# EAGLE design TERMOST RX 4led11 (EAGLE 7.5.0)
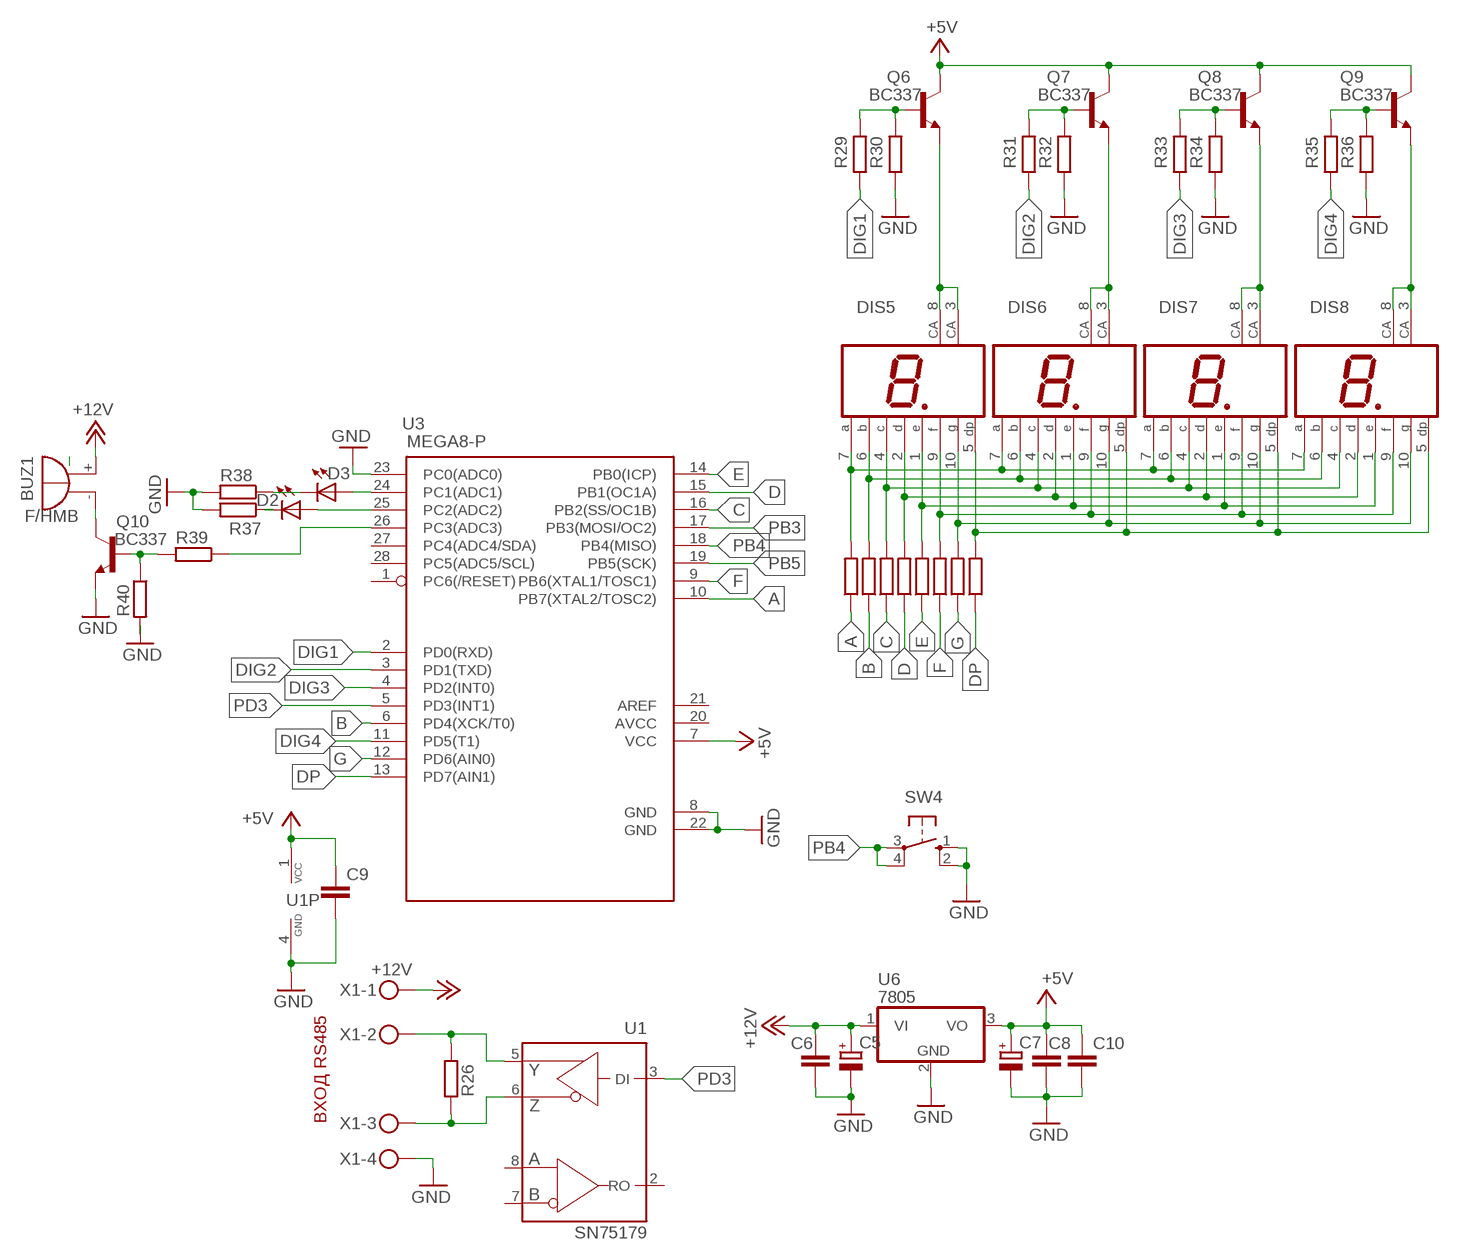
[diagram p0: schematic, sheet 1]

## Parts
BUZ1  F/HMB  [F/HMB]
C5  CPOL-EUE2.5-5  [E2,5-5]
C6  C-EUC1206  [C1206]
C7  CPOL-EUE2.5-5  [E2,5-5]
C8  C-EUC1206  [C1206]
C9  C-EUC1206  [C1206]
C10  C-EUC1206  [C1206]
D2  LED5MM  [LED5MM]
D3  LED5MM  [LED5MM]
DIS5  HD-H101  [HDSP-M]
DIS6  HD-H101  [HDSP-M]
DIS7  HD-H101  [HDSP-M]
DIS8  HD-H101  [HDSP-M]
Q6  BC337  [TO92]
Q7  BC337  [TO92]
Q8  BC337  [TO92]
Q9  BC337  [TO92]
Q10  BC337  [TO92]
R9  R-EU_0204/7  [0204/7]
R10  R-EU_0204/7  [0204/7]
R11  R-EU_0204/7  [0204/7]
R12  R-EU_0204/7  [0204/7]
R13  R-EU_0204/7  [0204/7]
R14  R-EU_0204/7  [0204/7]
R15  R-EU_0204/7  [0204/7]
R16  R-EU_0204/7  [0204/7]
R26  R-EU_0204/7  [0204/7]
R29  R-EU_0204/7  [0204/7]
R30  R-EU_0204/7  [0204/7]
R31  R-EU_0204/7  [0204/7]
R32  R-EU_0207/12  [0207/12]
R33  R-EU_0204/7  [0204/7]
R34  R-EU_0204/7  [0204/7]
R35  R-EU_0204/7  [0204/7]
R36  R-EU_0204/7  [0204/7]
R37  R-EU_0204/7  [0204/7]
R38  R-EU_0204/7  [0204/7]
R39  R-EU_0204/7  [0204/7]
R40  R-EU_0204/7  [0204/7]
SW4  10-XX  [B3F-10XX]
U1  SN75179  MAX488CPD  [DIL08]
U3  MEGA8-P  [DIL28-3]
U6  7805  7805T  [TO220H]
X1  MKDSN1,5/4-5,08  [MKDSN1,5/4-5,08]

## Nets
+5V: C7.+ C8.1 C9.1 C10.1 Q6.3(C) Q7.3(C) Q8.3(C) Q9.3(C) U1.1(VCC) U3.7(VCC) U6.3(VO)
+12V: BUZ1.+ C5.+ C6.1 U6.1(VI) X1.1
A: R9.1 U3.10(PB7(XTAL2/TOSC2))
B: R10.1 U3.6(PD4(XCK/T0))
C: R11.1 U3.16(PB2(SS/OC1B))
D: R12.1 U3.15(PB1(OC1A))
DIG1: R29.1 U3.2(PD0(RXD))
DIG2: R31.1 U3.3(PD1(TXD))
DIG3: R33.1 U3.4(PD2(INT0))
DIG4: R35.1 U3.11(PD5(T1))
DP: R16.1 U3.13(PD7(AIN1))
E: R13.1 U3.14(PB0(ICP))
F: R14.1 U3.9(PB6(XTAL1/TOSC1))
G: R15.1 U3.12(PD6(AIN0))
GND: C5.- C6.2 C7.- C8.2 C9.2 C10.2 Q10.1(E) R30.1 R32.1 R34.1 R36.1 R37.2 R38.2 R40.2 SW4.1(S) SW4.2(S1) U1.4(GND) U3.8(GND) U3.22(GND) U3.23(PC0(ADC0)) U6.2(GND) X1.4
N$1: DIS5.7(A) DIS6.7(A) DIS7.7(A) DIS8.7(A) R9.2
N$2: DIS5.6(B) DIS6.6(B) DIS7.6(B) DIS8.6(B) R10.2
N$3: DIS5.4(C) DIS6.4(C) DIS7.4(C) DIS8.4(C) R11.2
N$4: DIS5.2(D) DIS6.2(D) DIS7.2(D) DIS8.2(D) R12.2
N$5: DIS5.1(E) DIS6.1(E) DIS7.1(E) DIS8.1(E) R13.2
N$6: DIS5.9(F) DIS6.9(F) DIS7.9(F) DIS8.9(F) R14.2
N$7: DIS5.10(G) DIS6.10(G) DIS7.10(G) DIS8.10(G) R15.2
N$8: DIS5.5(DP) DIS6.5(DP) DIS7.5(DP) DIS8.5(DP) R16.2
N$9: DIS5.3(CA) DIS5.8(CA) Q6.1(E)
N$10: DIS6.3(CA) DIS6.8(CA) Q7.1(E)
N$11: Q6.2(B) R29.2 R30.2
N$12: Q7.2(B) R31.2 R32.2
N$13: DIS7.3(CA) DIS7.8(CA) Q8.1(E)
N$14: DIS8.3(CA) DIS8.8(CA) Q9.1(E)
N$15: Q8.2(B) R33.2 R34.2
N$16: Q9.2(B) R35.2 R36.2
N$17: BUZ1.- Q10.3(C)
N$18: Q10.2(B) R39.2 R40.1
N$19: R39.1 U3.26(PC3(ADC3))
N$20: D3.A U3.24(PC1(ADC1))
N$21: D2.A U3.25(PC2(ADC2))
N$23: D3.K(C) R38.1
N$25: D2.K(C) R37.1
N$26: R26.1 U1.5(Y) X1.2
N$27: R26.2 U1.6(Z) X1.3
PB3: U3.17(PB3(MOSI/OC2))
PB4: SW4.3(P) SW4.4(P1) U3.18(PB4(MISO))
PB5: U3.19(PB5(SCK))
PD3: U1.3(DI) U3.5(PD3(INT1))
Unconnected: U1.2(RO) U1.7(B) U1.8(A) U3.1(PC6(/RESET)) U3.21(AREF) U3.27(PC4(ADC4/SDA)) U3.28(PC5(ADC5/SCL))

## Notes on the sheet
- ВХОД RS485

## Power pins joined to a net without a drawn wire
AVCC: U3.20(AVCC)

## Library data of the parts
BUZ1 = buzzer:F/HMB: BUZZER; OC_FARNELL: unknown; OC_NEWARK: unknown
C5 C7 = rcl:CPOL-EU: POLARIZED CAPACITOR, European symbol
C6 C8-C10 = rcl:C-EU: CAPACITOR, European symbol
D2 D3 = led:LED: LED
DIS5-DIS8 = display-hp:HD-H101: LED DISPLAY 1-character 7 segment, decimal point right; OC_FARNELL: unknown; OC_NEWARK: unknown
Q6-Q10 = transistor:BC337: NPN TRANSISTOR
R9-R16 R26 R29-R40 = rcl:R-EU_: RESISTOR, European symbol
SW4 = switch-omron:10-XX: OMRON SWITCH; MPN: B3F-1000; OC_FARNELL: 176432; OC_NEWARK: 36M3542
U1 = maxim:MAX488: RS485 TRANSEIVER Source: Data sheet; OC_FARNELL: unknown; OC_NEWARK: unknown
U3 = atmel:MEGA8-P: MICROCONTROLLER 8 Kbytes FLASH, 1 kbytes SRAM, 512 bytes EEPROM, USART, 4-channel 10 bit ADC, 2-channel 8 bit ADC Pin compatible with Atmega48, ATMega88, ATMega168 Source: avr.lbr; OC_FARNELL: unknown; OC_NEWARK: unknown
U6 = linear:78*: Positive VOLTAGE REGULATOR Source: http://cache.national.com/ds/LM/LM78L05.pdf http://www.fairchildsemi.com/ds/LM/LM7805.pdf
X1 = con-phoenix-508:MKDSN1,5/4-5,08: MKDSN 1,5/ 4-5,08 Printklemme Nennstrom: 13,5 A Nennspannung: 250 V Rastermaß: 5,08 mm Polzahl: 4 Anschlussart: Schraubanschluss Montage: Löten Anschlussrichtung Leiter/Platine: 0 ° Artikelnummer: 1729144 Source: http://eshop.phoenixcontact.com .. 1729144.pdf

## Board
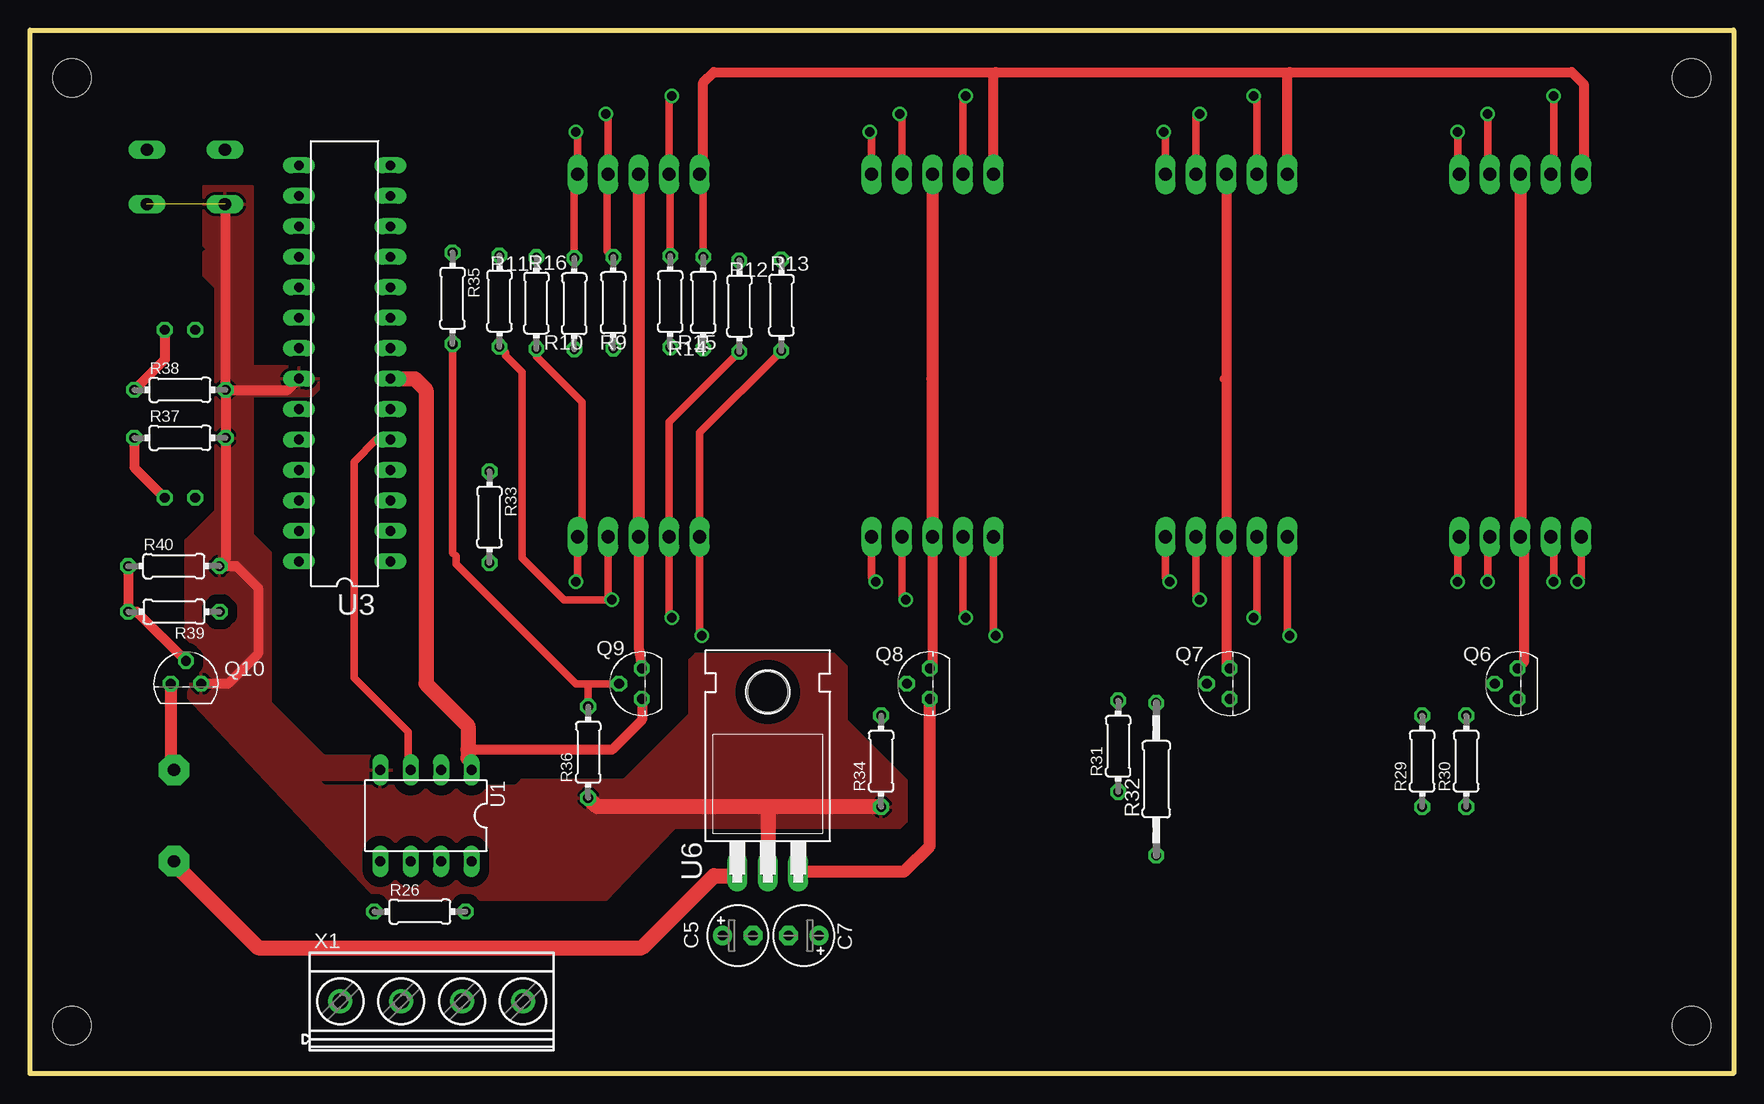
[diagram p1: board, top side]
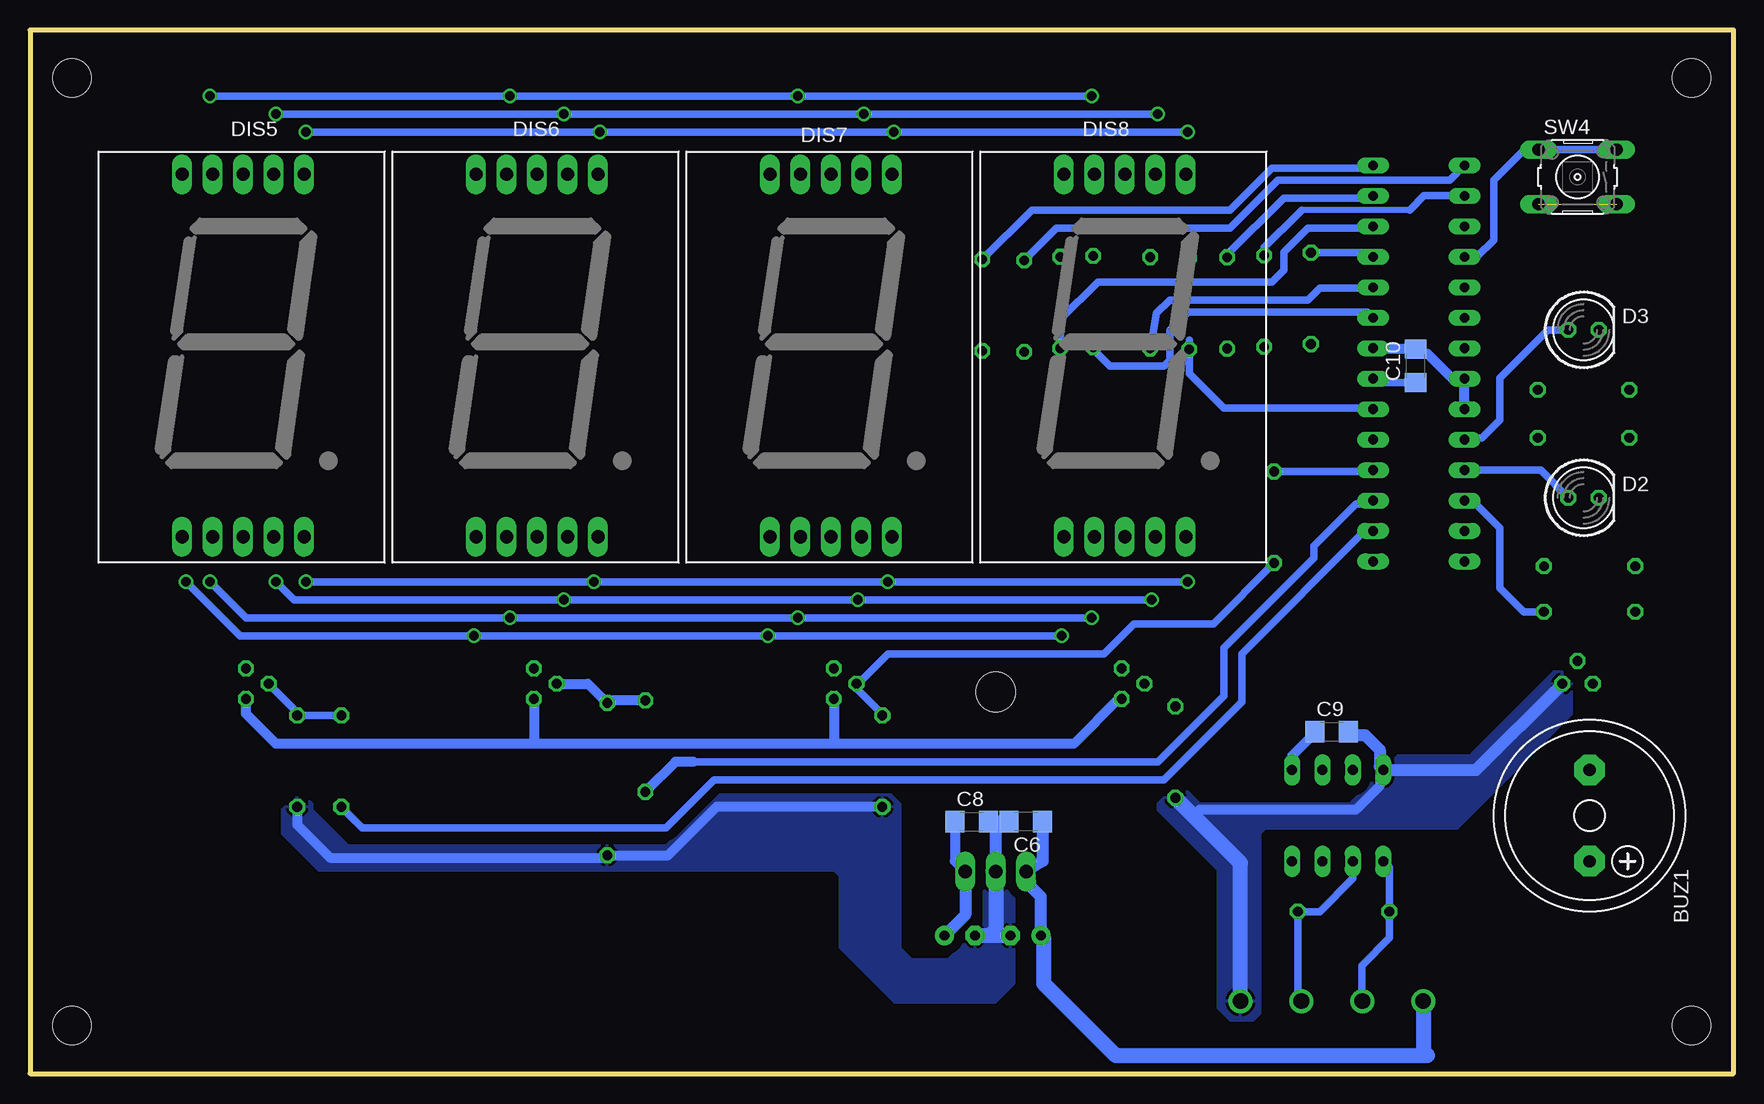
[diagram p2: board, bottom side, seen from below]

Size 142 x 87 mm. Coordinates in mm from the lower left corner, seen from the top.
Outline: 0,0 0,87 142,87 142,0 0,0
Copper layers (1*16): Top 0.035mm / dielectric 1.5mm / Bottom 0.035mm
Design rules "default": minimum track width 10mil, minimum drill 24mil, track to track 8mil, track to pad 8mil, pad to pad 8mil, via to via 8mil, smd to smd 8mil, copper to edge 40mil, drill to drill 8mil, minimum pad ring 10mil, minimum via ring 8mil, stop-mask expansion 4mil, vias tented up to drill 0mil, thermal gap 10mil
Holes 3.2 mm at 3.5,4 3.5,83 138.5,83 138.5,4

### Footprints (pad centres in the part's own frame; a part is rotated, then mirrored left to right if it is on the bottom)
F/HMB = drill 1.016 pad 2.54 octagon: + 3.81,0; - -3.81,0
E2,5-5 = drill 0.813 pad 1.6: + -1.27,0 | drill 0.813 pad 1.6 octagon: - 1.27,0
C1206 = smd 1.6 x 1.8: 1 -1.4,0; 2 1.4,0
LED5MM = drill 0.813 octagon: A -1.27,0; K 1.27,0
HDSP-M = drill 1.1 long: 1 -4.318,-16.256; 2 -1.778,-16.256; 3 0.762,-16.256; 4 3.302,-16.256; 5 5.842,-16.256; 6 5.842,13.97; 7 3.302,13.97; 8 0.762,13.97; 9 -1.778,13.97; 10 -4.318,13.97
TO92 = drill 0.813 octagon: 1 1.27,0; 2 0,1.905; 3 -1.27,0
0204/7 = drill 0.813 octagon: 1 -3.81,0; 2 3.81,0
0207/12 = drill 0.813 octagon: 1 -6.35,0; 2 6.35,0
B3F-10XX = drill 1.016 long: 1 -3.251,2.261; 2 3.251,2.261; 3 -3.251,-2.261; 4 3.251,-2.261
DIL08 = drill 0.813 long: 1 -3.81,-3.81; 2 -1.27,-3.81; 3 1.27,-3.81; 4 3.81,-3.81; 5 3.81,3.81; 6 1.27,3.81; 7 -1.27,3.81; 8 -3.81,3.81
DIL28-3 = drill 0.813 long: 1 -16.51,-3.81; 2 -13.97,-3.81; 3 -11.43,-3.81; 4 -8.89,-3.81; 5 -6.35,-3.81; 6 -3.81,-3.81; 7 -1.27,-3.81; 8 1.27,-3.81; 9 3.81,-3.81; 10 6.35,-3.81; 11 8.89,-3.81; 12 11.43,-3.81; 13 13.97,-3.81; 14 16.51,-3.81; 15 16.51,3.81; 16 13.97,3.81; 17 11.43,3.81; 18 8.89,3.81; 19 6.35,3.81; 20 3.81,3.81; 21 1.27,3.81; 22 -1.27,3.81; 23 -3.81,3.81; 24 -6.35,3.81; 25 -8.89,3.81; 26 -11.43,3.81; 27 -13.97,3.81; 28 -16.51,3.81
TO220H = drill 1.118 long: 1 -2.54,-10.16; 2 0,-10.16; 3 2.54,-10.16 | hole 3.302: 0,4.826
MKDSN1,5/4-5,08 = drill 1.3 pad 2: 1 -7.641,0.025; 2 -2.561,0.025; 3 2.519,0.025; 4 7.599,0.025

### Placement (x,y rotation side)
BUZ1  12,21.5 270 bottom
C5  59,11.5 0 top
C6  59,21 180 bottom
C7  64.5,11.5 180 top
C8  63.5,21 0 bottom
C9  33.5,28.5 0 bottom
C10  26.5,59 90 bottom
D2  12.5,48 0 bottom
D3  12.5,62 0 bottom
DIS5  125,61 0 bottom
DIS6  100.5,61 0 bottom
DIS7  76,61 0 bottom
DIS8  51.5,61 0 bottom
Q6  124,32.5 90 top
Q7  100,32.5 90 top
Q8  75,32.5 90 top
Q9  51,32.5 90 top
Q10  13,32.5 0 top
R9  48.62,64.26 90 top
R10  45.37,64.18 90 top
R11  39.13,64.4 270 top
R12  59.13,63.98 270 top
R13  62.63,64.06 270 top
R14  53.37,64.36 90 top
R15  56.12,64.28 90 top
R16  42.21,64.24 270 top
R26  32.5,13.5 0 top
R29  116.05,26.04 90 top
R30  119.72,26.04 90 top
R31  90.71,27.29 90 top
R32  93.88,24.54 90 top
R33  38.3,46.38 270 top
R34  70.95,26.04 90 top
R35  35.22,64.63 270 top
R36  46.53,26.79 90 top
R37  12.5,53 0 top
R38  12.5,57 0 top
R39  12,38.5 180 top
R40  11.99,42.3 0 top
SW4  13,74.75 180 bottom
U1  33,21.5 180 top
U3  26.23,59.2 90 top
U6  61.5,27 0 top
X1  33.5,6 0 top

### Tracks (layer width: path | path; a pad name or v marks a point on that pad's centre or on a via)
+5V
  Top 0.813: Q9.3 51,29.5 48.5,27 36.5,27
  Top 1.016: U6.3 72.84,16.84 75,19 Q8.3
  Top 1.27: U3.7 32.07,57.93 33,57 33,32.5 36.5,29 36.5,27 36.5,26.31 36.81,26 U1.1
  Bottom 0.61: C10.1 29.71,57.6 U3.7
  Bottom 0.813: Q9.3 51.27,31.23 55,27.5 75,27.5 | 75,27.5 100,27.5 | 100,27.5 121.5,27.5 124,30 Q6.3 | Q7.3 100,27.5 | Q8.3 75,27.5 | C9.1 34.9,28.41 36.81,26.5 U1.1 | C8.1 64.9,17.7 U6.3
  Bottom 1.016: U6.3 64.04,13.23 C7.+
+12V
  Top 1.27: 58.8,17 U6.1 58.62,16.5 57,16.5 51,10.5 19,10.5 12,17.5 BUZ1.+
  Bottom 1.016: C6.1 57.6,17.7 U6.1 59,16.3 59,16 57.73,14.73 C5.+
  Bottom 1.27: X1.1 25.86,1.86 25.5,1.5 51.5,1.5 57.5,7.5 57.5,11.27 C5.+
A
  Bottom 0.61: R9.1 48.12,63.38 47,64.5 35.5,64.5 34.5,65.5 30.09,65.5 U3.10
B
  Bottom 0.61: 45.37,61.13 R10.1 45.37,58.37 42.5,55.5 30.15,55.5 U3.6
C
  Bottom 0.5: 27,72 36,72
  Bottom 0.61: R11.1 39.13,68.87 36.25,71.75 36,72 | U3.16 25.83,73.17 27,72
D
  Bottom 0.61: U3.15 23.63,74.5 38,74.5 42,70.5 56.42,70.5 R12.1
DIG1
  Bottom 0.61: U3.2 30.77,45.23 41,35 41,31 47.5,24.5 85,24.5 89,20.5 114.32,20.5 R29.1
DIG2
  Bottom 0.61: U3.3 30.31,47.5 31.5,47.5 35,44 35,43 42.5,35.5 42.5,31.5 48,26 86.69,26
  Bottom 0.813: 86.69,26 88.19,26 R31.1
DIG3
  Bottom 0.61: R33.1 30.16,50.19 U3.4
DIG4
  Bottom 0.61: R35.1 30.39,68.44 U3.11
DP
  Bottom 0.61: R16.1 42.21,68.29 37.5,73 30.21,73 U3.13
E
  Bottom 0.61: U3.14 30.25,75.5 38.5,75.5 42,72 58.5,72 R13.1
F
  Bottom 0.61: R14.1 53.37,60.37 52,59 47.5,59 47,59.5 47,62 45.5,63.5 30.53,63.5 U3.9
G
  Bottom 0.61: R15.1 56.12,62.88 53,66 38.5,66 37.5,67 37.5,68.5 35.5,70.5 30.17,70.5 U3.12
GND  (1 unrouted)
  Top 0.813: SW4.2 16.25,57.06 R38.2 | R38.2 R37.2 16.31,42.81 R40.2 17.2,42.3 19,40.5 19,35 16.5,32.5 Q10.1 | R38.2 21.49,57 U3.22
  Top 1.27: R36.1 47.28,22.23 R34.1 61.73,22.23 61.5,22 U6.2
  Bottom 0.813: R34.1 84.77,22.23 88.81,18.19 R32.1 94.07,18 117,18 119.72,20.72 R30.1 | U3.23 U3.22 23.43,57.93 25.5,60 26.1,60 C10.2 29.97,60.4 U3.8 | 29.5,27 29.5,24 31.5,22 44.5,22 45.02,21.48
  Bottom 1.016: C9.2 32.1,28.22 30.72,28.22 29.5,27 29.5,25.62 U1.4 21.46,25.31 Q10.1 | C6.2 61.5,21 | 61.5,21 C8.2 | U6.2 61.5,21
  Bottom 1.27: C5.- 62,11.5 | 62,11.5 C7.- | U6.2 61.5,12 62,11.5 | X1.4 41.1,17.55 45.02,21.48 R36.1
  pour Bottom (isolate 0.813): 13.5,33.5 15,33.5 22,26.5 28,26.5 32,22.5 44.5,22.5 45.5,23.5 47,23.5 48,22.5 48,22 43,17 43,5.5 42,4.5 40,4.5 39.5,5 39.5,20 39,20.5 23,20.5 13.5,30
  pour Top (isolate 0.813): 44.5,24.5 49.5,24.5 55,30 55,34.5 55.5,35 67,35 68,34 68,29.5 73,24.5 73,21 72.5,20.5 45,20.5 43.5,22 43.5,23.5
  pour Top (isolate 0.813): 48,14.5 29,14.5 13,31.5 13,42 15.5,44.5 15.5,65.5 14.5,66.5 14.5,68.5 15,69 18,69 18.5,68.5 18.5,42.5 20,41 20,28.5 24.5,24 40.5,24 41,24.5 57.5,24.5
  pour Bottom (isolate 0.813): 61.5,18 62,18 62.5,17.5 62.5,12.5 64.5,10.5 65.5,9.5 68.5,9.5 69.5,10.5 69.5,22.5 70.5,23.5 84.5,23.5 89,19 115.5,19 118.5,22 118.5,22.5 119,23 120,23 121,22 121,20 118,17 75,17 74.5,16.5 74.5,10.5 70,6 61.5,6 60.5,7 60,7.5 60,17.5 60.5,18
  pour Top (isolate 0.813): 18.5,59 23.5,59 24,58.5 24,57 23.5,56.5 18.5,56.5
  pour Top (isolate 0.813): 43.5,24.5 22.5,24.5 13,34 13,44.5 15.5,47 15.5,68 14.5,69 14.5,74 18.5,74 18.5,45 20,43.5 20,31 24.5,26.5 40.5,26.5 41,27 44.5,27 44.5,25.5
N$1  (via drill 0.8)
  Top 0.61: v48,80 48.2,79.8 DIS8.7 48.12,74.89 48.12,68.57 R9.2 | v121.5,80 121.5,75.17 DIS5.7 | DIS7.7 72.7,79.8 v72.5,80 | DIS6.7 97.2,79.7 v97.5,80
  Top 0.813: 121.62,74.89 DIS5.7
  Bottom 0.61: v48,80 v72.5,80 v97.5,80 v121.5,80
N$2  (via drill 0.8)
  Top 0.61: v45.5,78.5 45.66,78.34 DIS8.6 45.37,74.68 R10.2 | v119,78.5 119,75.13 DIS5.6 | DIS7.6 70.16,78.34 v70,78.5 | DIS6.6 94.66,78.34 v94.5,78.5
  Bottom 0.61: v45.5,78.5 v70,78.5 v94.5,78.5 v119,78.5
N$3  (via drill 0.8)
  Top 0.61: DIS8.4 48.2,39.8 v48.5,39.5 44.5,39.5 41,43 41,58.5 39.63,59.87 39.63,60.09 R11.2 | DIS5.4 121.5,44.55 v121.5,41 121.37,40.87 | DIS7.4 72.7,39.8 v73,39.5 | DIS6.4 97.2,39.8 v97.5,39.5
  Bottom 0.61: v48.5,39.5 v73,39.5 v97.5,39.5 120,39.5 v121.5,41
N$4  (via drill 0.8)
  Top 0.61: DIS6.2 102.28,38.28 v102,38 | v53.5,38 53.28,38.22 DIS8.2 53.28,54.32 R12.2 | DIS7.2 77.78,38.22 v78,38 | v127,41 127,44.52 DIS5.2
  Bottom 0.61: v53.5,38 v78,38 v102,38 124,38 v127,41
N$5  (via drill 0.8)
  Top 0.61: DIS6.1 104.82,36.68 v105,36.5 | v56,36.5 55.82,36.68 DIS8.1 55.82,53.44 R13.2 | DIS7.1 80.32,36.68 v80.5,36.5 | DIS5.1 129.32,41.32 v129,41
  Bottom 0.61: v56,36.5 v80.5,36.5 v105,36.5 124.5,36.5 v129,41
N$6  (via drill 0.8)
  Top 0.61: v53.5,81.5 53.28,81.28 DIS8.9 53.37,74.88 R14.2 | v127,81.5 127,75.19 DIS5.9 | DIS7.9 77.78,81.28 v78,81.5 | DIS6.9 102.28,81.22 v102,81.5
  Top 0.813: 126.87,74.88 DIS5.9
  Bottom 0.61: v53.5,81.5 v78,81.5 v102,81.5 v127,81.5
N$7
  Top 0.61: R15.2 56.12,74.67 DIS8.10
  Top 0.813: 56.12,74.67 56.12,82.62 57,83.5 80.5,83.5 | 80.5,83.5 105,83.5 | 105,83.5 128.5,83.5 129.5,82.5 129.5,75.15 DIS5.10 | DIS7.10 80.32,83.32 80.5,83.5 | DIS6.10 104.82,83.32 105,83.5
N$8  (via drill 0.8)
  Top 0.61: v45.5,41 45.66,41.16 DIS8.5 46,45.09 46,56 42.21,59.79 R16.2 | v119,41 119,44.59 DIS5.5 | DIS7.5 70.16,41.34 v70.5,41 | DIS6.5 94.66,41.34 v95,41
  Bottom 0.61: v45.5,41 v70.5,41 v95,41 v119,41 | DIS8.5 45.26,44.74
N$9
  Top 0.61: 124.5,44.48 DIS5.3 | 124.14,57.9 124.24,58
  Top 0.813: 124.5,44.48 124.5,34.27 Q6.1
  Top 1.016: DIS5.8 124.24,58 DIS5.3
N$10
  Top 0.813: DIS6.8 99.74,57.75 | 99.74,57.75 DIS6.3 99.74,34.03 Q7.1 | 99.59,57.9 99.74,57.75
N$11
  Bottom 0.61: R29.2 R30.2 119.72,30.12 Q6.2
  Bottom 0.813: 122.05,32.45 Q6.2
N$12
  Bottom 0.813: R31.2 93.67,31.1 R32.2 95.49,32.5 Q7.2
N$13
  Top 0.61: 75.25,45.24 75.24,45.25
  Top 0.813: 75.14,57.9 75.24,58 | DIS7.3 75.24,34.01 Q8.1
  Top 1.016: DIS7.8 75.24,58 75.24,45.25 DIS7.3
N$14
  Top 0.813: DIS8.3 50.74,35.53 Q9.1
  Top 1.016: DIS8.8 DIS8.3
N$15
  Bottom 0.61: R33.2 43.37,37.5 50,37.5 52.5,35 70.5,35 73,32.5 Q8.2 73,32.41 73,32 70.95,29.95 R34.2
N$16
  Top 0.61: R35.2 35.22,43.41 35.5,43.13 35.5,42.5 45.5,32.5 46.5,32.5 | Q9.2 46.5,32.5 | R36.2 46.53,32.47 46.5,32.5
N$17
  Top 1.016: Q10.3 11.73,25.58 BUZ1.-
N$18
  Top 0.813: R40.1 R39.2 8.9,38.5 Q10.2
N$19
  Bottom 0.61: U3.26 21.77,47.77 19.5,45.5 19.5,40.5 17.5,38.5 R39.1
N$20
  Bottom 0.61: D3.A 15.5,62 19.5,58 19.5,54.5 21,53 22.27,53 U3.24
N$21
  Bottom 0.61: U3.25 16.08,50.31 D2.A
N$23
  Top 0.813: D3.K 11.23,59.54 R38.1
N$25
  Top 0.813: R37.1 8.69,50.54 D2.K
N$26
  Bottom 0.61: U1.5 28.69,17.19 R26.1 28.69,11.31 31,9 31,6.09 X1.2
N$27
  Bottom 0.61: X1.3 36.31,6.32 R26.2 34.5,13.5 31.73,16.27 U1.6
PB4
  Bottom 0.61: U3.18 21.41,68.09 20,69.5 20,74.5 17.5,77 16.26,77 SW4.4 SW4.3
PD3
  Top 0.61: U3.5 28.85,52.85 27,51 27,33 31.5,28.5 31.5,25.54
  Top 0.813: 31.5,25.54 U1.3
